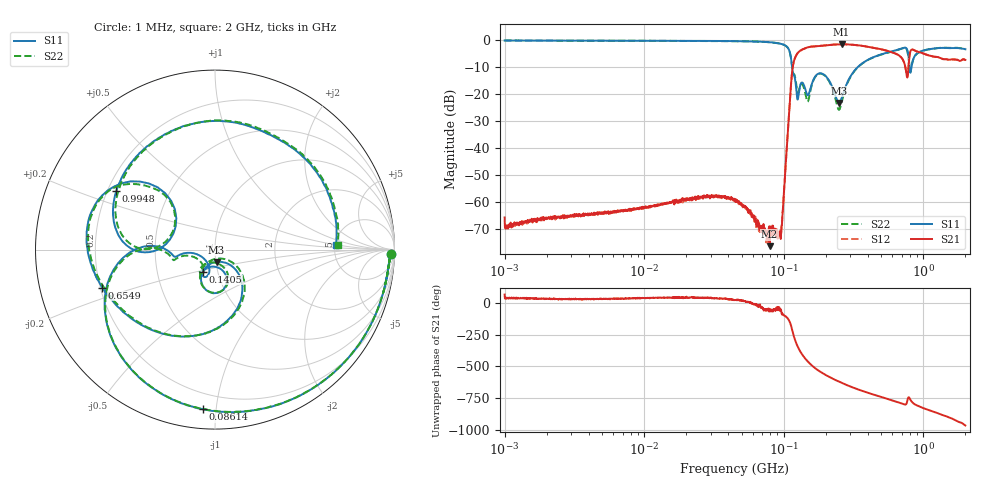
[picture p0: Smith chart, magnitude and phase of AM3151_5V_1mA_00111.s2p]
! Date/Time: Fri Jun 26 10:34:47 2020
! Network Analyzer:  Rev:
! Sweep from 1000000.0 to 2000000000.0, 1601 Points ! Power Supply: 0 V, 0 A
# HZ S DB R 50
!freq MagS11 AngS11 MagS21 AngS21 MagS12 AngS12 MagS22 AngS22
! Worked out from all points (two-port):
!   1601 points, 1 MHz to 2 GHz, reference 50 ohm
!   highest |S21| = -1.55 dB at 259.3 MHz (marker M1); lowest = -76.2 dB at 79.08 MHz (marker M2)
!   |S21| within 3 dB of the highest: 127.1 MHz to 596.4 MHz (469.4 MHz wide, 130 % of centre); 803.4 MHz to 945.6 MHz (142.2 MHz wide, 16.3 % of centre)
!   lowest |S11| = -23.2 dB at 248.5 MHz (marker M3), VSWR 1.15, Z = 50.4 - j6.93 ohm
!   |S11| at or under -10 dB: 114.6 MHz to 338.7 MHz (224.1 MHz wide, 98.9 % of centre); 795.8 MHz to 821.9 MHz (26.11 MHz wide, 3.23 % of centre)
!   |S22| runs from -25.8 to -0.2 dB; largest |S21 - S12| = 0.0096
!   S11 on the Smith chart (normalised r, x): 1 MHz: 38, -52; 86.14 MHz: 0.11, -0.92; 140.5 MHz: 0.85, -0.21; 654.9 MHz: 0.21, -0.16; 994.8 MHz: 0.24, +0.26; 2 GHz: 5.10, +0.49
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1000000  -0.16 -1.4  -65.62 67.2  -69.07 38.3  -0.16 -1.5
3555161  -0.23 -3.7  -64.64 32.4  -64.44 30.1  -0.23 -3.7
1.263916e7  -0.28 -11.9  -61.01 41.5  -60.98 41.8  -0.28 -11.8
4.493426e7  -0.40 -42.8  -59.80 24.1  -59.39 27.5  -0.41 -42.7
7.908452e7  -0.80 -83.2  -76.23 -51.4  -71.69 -44.6  -0.81 -83.1
8.614461e7  -0.99 -94.3  -69.71 -50.4  -70.61 -60.0  -1.00 -94.2
9.6548e7  -1.47 -114.9  -68.39 -84.5  -68.86 -76.4  -1.48 -114.8
1.167534e8  -12.47 -172.9  -9.04 116.5  -9.04 116.5  -12.22 -169.1
1.283903e8  -19.21 -106.9  -4.30 -3.8  -4.31 -3.9  -18.53 -122.7
1.405178e8  -17.13 -118.2  -3.14 -70.5  -3.14 -70.5  -18.31 -128.0
1.589914e8  -16.14 -67.1  -2.42 -133.4  -2.41 -133.6  -16.52 -62.2
1.904465e8  -12.54 -99.3  -2.10 164.5  -2.08 164.4  -12.61 -99.9
2.4849e8  -23.22 -82.7  -1.58 98.7  -1.59 98.8  -25.80 -81.6
2.593446e8  -21.55 -56.7  -1.55 89.5  -1.57 89.5  -23.13 -47.4
3.721142e8  -8.29 -76.6  -2.21 22.7  -2.21 22.6  -8.37 -74.1
5.652395e8  -4.50 -137.5  -4.15 -40.4  -4.14 -40.4  -4.55 -138.0
6.54923e8  -3.57 -161.4  -5.39 -62.5  -5.38 -62.6  -3.62 -162.8
7.552395e8  -3.00 157.1  -12.17 -76.4  -12.20 -76.1  -3.23 153.9
8.148812e8  -11.25 173.4  -3.74 -51.2  -3.74 -51.1  -11.09 170.9
9.948255e8  -3.88 149.4  -4.92 -109.3  -4.89 -108.9  -3.93 146.5
1.413901e9  -2.90 82.5  -7.07 -169.1  -7.05 -169.1  -2.84 79.5
2e9  -3.42 2.2  -7.32 112.9  -7.46 112.4  -3.30 1.9
